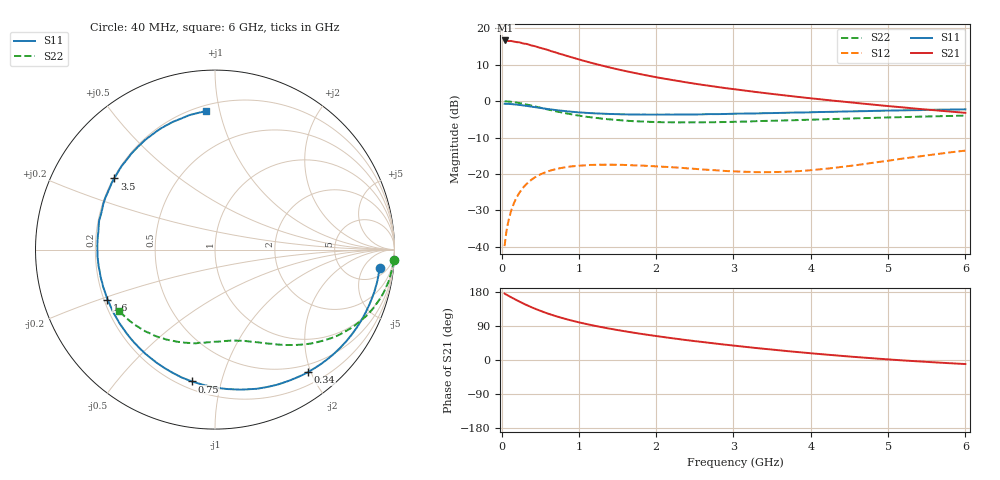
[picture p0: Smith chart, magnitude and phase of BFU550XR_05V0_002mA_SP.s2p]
! Filename:  P:\Prog\Test\Noise\ATS_data\Testdata_Net\03 Spar\BFU550XR_APG2013_45_C05_05p0V_002mA_SP_CM01_D.s2p
! Date/Time: Tue 06/Aug/2013 14:38:15
! BFU550XR_APG2013_45_C05_05p0V_1to35mA_SP_CM01_Bias2_R.s2p
! MDIF S-parameter v. bias file
! BFU550XR_APG2013_45_C05_05p0V_1to35mA_SP_CM01
! Date/time Fri Aug 02 14:46:46 2013
! VAR V_out= 5.0000
! VAR I_out= 2.0000
! VAR V_in= 0.7931
! VAR I_in= 0.0216
! Device data file deembeded for feedlines and parallel
! Original file: \03 Spar\BFU550XR_APG2013_45_C05_05p0V_002mA_SP_CM01_R.s2p
! Feed-files: PR006V01_02082013_Feed1.s2p, PR006V01_02082013_Feed2.s2p
! Parallel-file: PR006V01_02082013_Par.s2p
# MHz S MA R 50
!  Freq-MHz  S11-mag  S11-arg  S21-mag  S21-arg  S12-mag  S12-arg  S22-mag  S22-arg
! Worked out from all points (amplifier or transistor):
!   98 points, 40 MHz to 6 GHz, reference 50 ohm
!   highest |S21| = 16.7 dB at 50 MHz (marker M1)
!   |S21| within 3 dB of that: start of sweep to 651.8 MHz
!   unconditionally stable (mu >= 1): 3.058 GHz to 4.655 GHz
!   at 300 MHz: K = 0.10, MSG = 19.5 dB, |S12| = -23.2 dB
!   at 1.6 GHz: K = 0.50, MSG = 12.9 dB, |S12| = -17.5 dB
!   at 6 GHz: K = 0.80, MSG = 5.2 dB, |S12| = -13.6 dB
!   S11 on the Smith chart (normalised r, x): 40 MHz: 8, -12; 340 MHz: 0.38, -1.96; 750 MHz: 0.24, -0.81; 1.6 GHz: 0.21, -0.21; 3.5 GHz: 0.20, +0.31; 6 GHz: 0.24, +0.91
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40  0.924 -6.5  6.81 175.5  0.01024 86.1  0.9964 -3.4
50  0.9222 -8.1  6.817 173.6  0.01276 85.0  0.9957 -4.4
60  0.9217 -9.8  6.757 172.9  0.01532 84.2  0.9946 -5.3
120  0.9131 -19.5  6.713 166.1  0.03017 78.2  0.9829 -10.6
220  0.8918 -35.2  6.452 155.4  0.05291 69.1  0.9479 -18.8
320  0.8627 -50.0  6.124 145.4  0.0724 60.8  0.903 -26.2
340  0.8573 -52.8  6.04 143.6  0.0758 59.2  0.8931 -27.6
440  0.8264 -66.1  5.65 134.8  0.09113 52.2  0.8449 -33.7
550  0.7937 -79.5  5.226 126.1  0.104 45.3  0.7909 -39.8
600  0.7796 -85.1  5.045 122.5  0.1087 42.6  0.7687 -42.1
750  0.7457 -100.0  4.479 112.9  0.12 35.6  0.7106 -48.2
900  0.7172 -113.1  4.026 104.4  0.1273 29.8  0.6628 -53.3
1050  0.6974 -124.2  3.619 97.1  0.131 25.0  0.6215 -57.9
1300  0.6739 -139.9  3.083 86.5  0.1342 18.8  0.5764 -64.1
1600  0.6604 -155.1  2.599 75.7  0.1332 13.5  0.5414 -70.6
2050  0.6546 -173.2  2.087 61.9  0.1265 9.2  0.5156 -79.2
2500  0.6571 171.8  1.739 49.8  0.1179 8.2  0.5129 -87.3
3100  0.6756 154.8  1.42 35.9  0.108 13.2  0.5239 -97.8
3500  0.6871 144.8  1.259 27.5  0.1064 19.3  0.5388 -105.0
4100  0.7095 131.0  1.069 16.0  0.1156 29.4  0.5611 -115.3
5200  0.7495 108.3  0.8207 -1.2  0.1637 37.7  0.6052 -133.9
6000  0.7736 93.6  0.6925 -10.7  0.2098 35.4  0.6341 -147.2
